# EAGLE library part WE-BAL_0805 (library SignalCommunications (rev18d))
WE-BAL Multilayer Chip Balun Characteristics Low loss SMD Balun with balanced impedance of 50 to 200 Ω Operating temperature: –40 °C to +85 °C Power Capacity: 2 W max. Applications RF applications Wireless communication systems like Home RF, DECT, WLAN, Bluetooth, ZigBee … Details see: http://katalog.we-online.de/en/pbs/WE-BAL Updated by Dan Xu 2014-06-19 2014 (C) Wurth Elektronik
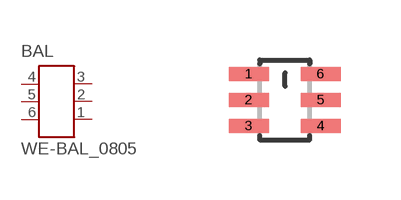
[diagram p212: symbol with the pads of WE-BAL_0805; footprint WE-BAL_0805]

Designator prefix BAL

## WE-BAL_0805_748421245, WE-BAL_0805_748421551, WE-BAL_0805_748422245, WE-BAL_0805_748425245  [WE-BAL_0805]
1  1  pas
2  2  pas
3  3  pas
4  4  pas
5  5  pas
6  6  pas

## Footprint WE-BAL_0805 (pad centres in mm)
Multilayer Chip Baluns WE-BAL
smd 1 x 0.35: 1 -0.9,0.65; 2 -0.9,0; 3 -0.9,-0.65; 4 0.9,-0.65; 5 0.9,0; 6 0.9,0.65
